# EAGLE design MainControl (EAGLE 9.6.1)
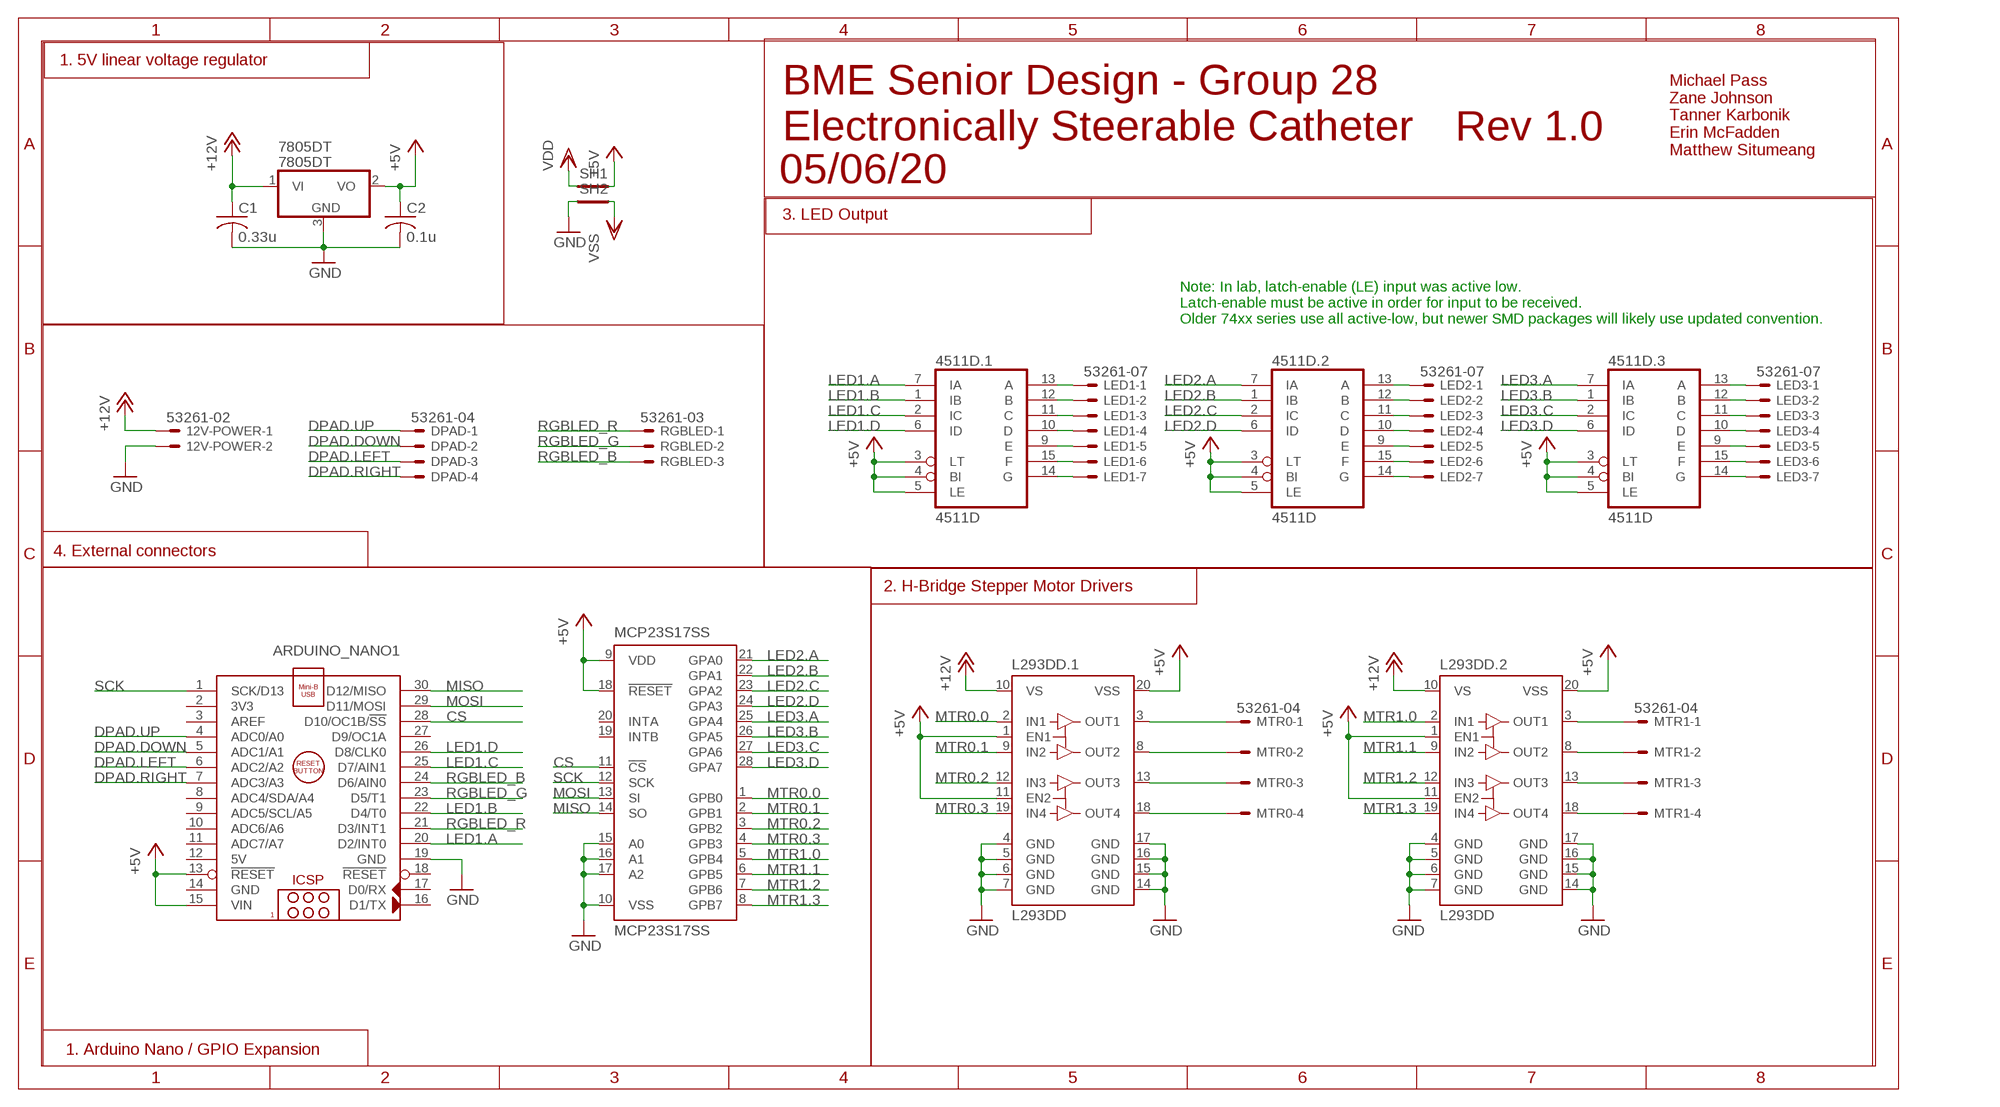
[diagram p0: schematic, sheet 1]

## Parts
12V-POWER  53261-02  [53261-02]
4511D.1  4511D  [SO16]
4511D.2  4511D  [SO16]
4511D.3  4511D  [SO16]
7805DT  7805DT  [TO252]
ARDUINO_NANO1  ARDUINO_NANO  [ARDUINO_NANO]
C1  0.33u  C-USC0805  [C0805]
C2  0.1u  C-USC0805  [C0805]
DPAD  53261-04  [53261-04]
L293DD.1  L293DD  [SO20]
L293DD.2  L293DD  [SO20]
LED1  53261-07  [53261-07]
LED2  53261-07  [53261-07]
LED3  53261-07  [53261-07]
MCP23S17SS  MCP23S17SS  [SSOP28]
MTR0  53261-04  [53261-04]
MTR1  53261-04  [53261-04]
RGBLED  53261-03  [53261-03]
SH1  SHORTT5  [SHORT_TOP-50]
SH2  SHORTT5  [SHORT_TOP-50]

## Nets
+5V: 4511D.1.3(LT) 4511D.1.4(BI) 4511D.1.5(LE) 4511D.2.3(LT) 4511D.2.4(BI) 4511D.2.5(LE) 4511D.3.3(LT) 4511D.3.4(BI) 4511D.3.5(LE) 7805DT.2(VO) ARDUINO_NANO1.13(!RESET) ARDUINO_NANO1.15(VIN) C2.1 L293DD.1.1(EN1) L293DD.1.11(EN2) L293DD.1.20(VSS) L293DD.2.1(EN1) L293DD.2.11(EN2) L293DD.2.20(VSS) MCP23S17SS.9(VDD) MCP23S17SS.18(!RESET) SH1.2
+12V: 12V-POWER.1 7805DT.1(VI) C1.1 L293DD.1.10(VS) L293DD.2.10(VS)
CS: ARDUINO_NANO1.28(D10/OC1B/!SS) MCP23S17SS.11(!CS)
DPAD.DOWN: ARDUINO_NANO1.5(ADC1/A1) DPAD.2
DPAD.LEFT: ARDUINO_NANO1.6(ADC2/A2) DPAD.3
DPAD.RIGHT: ARDUINO_NANO1.7(ADC3/A3) DPAD.4
DPAD.UP: ARDUINO_NANO1.4(ADC0/A0) DPAD.1
GND: 12V-POWER.2 7805DT.3(GND) ARDUINO_NANO1.19(GND) C1.2 C2.2 L293DD.1.4(GND) L293DD.1.5(GND) L293DD.1.6(GND) L293DD.1.7(GND) L293DD.1.14(GND) L293DD.1.15(GND) L293DD.1.16(GND) L293DD.1.17(GND) L293DD.2.4(GND) L293DD.2.5(GND) L293DD.2.6(GND) L293DD.2.7(GND) L293DD.2.14(GND) L293DD.2.15(GND) L293DD.2.16(GND) L293DD.2.17(GND) MCP23S17SS.10(VSS) MCP23S17SS.15(A0) MCP23S17SS.16(A1) MCP23S17SS.17(A2) SH2.1
LED1.A: 4511D.1.7(IA) ARDUINO_NANO1.20(D2/INT0)
LED1.B: 4511D.1.1(IB) ARDUINO_NANO1.22(D4/T0)
LED1.C: 4511D.1.2(IC) ARDUINO_NANO1.25(D7/AIN1)
LED1.D: 4511D.1.6(ID) ARDUINO_NANO1.26(D8/CLK0)
LED2.A: 4511D.2.7(IA) MCP23S17SS.21(GPA0)
LED2.B: 4511D.2.1(IB) MCP23S17SS.22(GPA1)
LED2.C: 4511D.2.2(IC) MCP23S17SS.23(GPA2)
LED2.D: 4511D.2.6(ID) MCP23S17SS.24(GPA3)
LED3.A: 4511D.3.7(IA) MCP23S17SS.25(GPA4)
LED3.B: 4511D.3.1(IB) MCP23S17SS.26(GPA5)
LED3.C: 4511D.3.2(IC) MCP23S17SS.27(GPA6)
LED3.D: 4511D.3.6(ID) MCP23S17SS.28(GPA7)
MISO: ARDUINO_NANO1.30(D12/MISO) MCP23S17SS.14(SO)
MOSI: ARDUINO_NANO1.29(D11/MOSI) MCP23S17SS.13(SI)
MTR0.0: L293DD.1.2(IN1) MCP23S17SS.1(GPB0)
MTR0.1: L293DD.1.9(IN2) MCP23S17SS.2(GPB1)
MTR0.2: L293DD.1.12(IN3) MCP23S17SS.3(GPB2)
MTR0.3: L293DD.1.19(IN4) MCP23S17SS.4(GPB3)
MTR1.0: L293DD.2.2(IN1) MCP23S17SS.5(GPB4)
MTR1.1: L293DD.2.9(IN2) MCP23S17SS.6(GPB5)
MTR1.2: L293DD.2.12(IN3) MCP23S17SS.7(GPB6)
MTR1.3: L293DD.2.19(IN4) MCP23S17SS.8(GPB7)
N$1: 4511D.1.13(A) LED1.1
N$2: 4511D.1.12(B) LED1.2
N$3: 4511D.1.11(C) LED1.3
N$12: 4511D.1.10(D) LED1.4
N$13: 4511D.1.9(E) LED1.5
N$14: 4511D.1.15(F) LED1.6
N$15: 4511D.1.14(G) LED1.7
N$16: 4511D.2.13(A) LED2.1
N$17: 4511D.2.12(B) LED2.2
N$18: 4511D.2.11(C) LED2.3
N$19: 4511D.2.10(D) LED2.4
N$20: 4511D.2.9(E) LED2.5
N$21: 4511D.2.15(F) LED2.6
N$22: 4511D.2.14(G) LED2.7
N$23: 4511D.3.13(A) LED3.1
N$24: 4511D.3.12(B) LED3.2
N$25: 4511D.3.11(C) LED3.3
N$26: 4511D.3.10(D) LED3.4
N$27: 4511D.3.9(E) LED3.5
N$28: 4511D.3.15(F) LED3.6
N$29: 4511D.3.14(G) LED3.7
N$30: L293DD.1.3(OUT1) MTR0.1
N$31: L293DD.1.8(OUT2) MTR0.2
N$32: L293DD.1.13(OUT3) MTR0.3
N$33: L293DD.1.18(OUT4) MTR0.4
N$34: L293DD.2.3(OUT1) MTR1.1
N$35: L293DD.2.8(OUT2) MTR1.2
N$36: L293DD.2.13(OUT3) MTR1.3
N$37: L293DD.2.18(OUT4) MTR1.4
RGBLED_B: ARDUINO_NANO1.24(D6/AIN0) RGBLED.3
RGBLED_G: ARDUINO_NANO1.23(D5/T1) RGBLED.2
RGBLED_R: ARDUINO_NANO1.21(D3/INT1) RGBLED.1
SCK: ARDUINO_NANO1.1(SCK/D13) MCP23S17SS.12(SCK)
VDD: SH1.1
VSS: SH2.2
Unconnected: ARDUINO_NANO1.2(3V3) ARDUINO_NANO1.3(AREF) ARDUINO_NANO1.8(ADC4/SDA/A4) ARDUINO_NANO1.9(ADC5/SCL/A5) ARDUINO_NANO1.10(ADC6/A6) ARDUINO_NANO1.11(ADC7/A7) ARDUINO_NANO1.16(D1/TX) ARDUINO_NANO1.17(D0/RX) ARDUINO_NANO1.18(!RESET) ARDUINO_NANO1.27(D9/OC1A) MCP23S17SS.19(INTB) MCP23S17SS.20(INTA)

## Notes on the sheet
- 1. 5V linear voltage regulator
- BME Senior Design - Group 28
- Electronically Steerable Catheter | Rev 1.0
- Michael Pass
  Zane Johnson
  Tanner Karbonik
  Erin McFadden
  Matthew Situmeang
- 05/06/20
- 3. LED Output
- Note: In lab, latch-enable (LE) input was active low. 
  Latch-enable must be active in order for input to be received. 
  Older 74xx series use all active-low, but newer SMD packages will likely use updated convention.
- 4. External connectors
- 2. H-Bridge Stepper Motor Drivers
- 1. Arduino Nano / GPIO Expansion

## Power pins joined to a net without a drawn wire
5V: ARDUINO_NANO1.12(5V)
GND: ARDUINO_NANO1.14(GND)
VDD: 4511D.1.16(VDD) 4511D.2.16(VDD) 4511D.3.16(VDD)
VSS: 4511D.1.8(VSS) 4511D.2.8(VSS) 4511D.3.8(VSS)

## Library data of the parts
12V-POWER = con-molex:53?-02: CONNECTOR; MF: MOLEX; OC_FARNELL: 1125373; OC_NEWARK: unknown
4511D.1-4511D.3 = 45xx:4511: BCD to 7-segment LATCH/DECODER/DRIVER
7805DT = linear:78*: Positive VOLTAGE REGULATOR Source: http://cache.national.com/ds/LM/LM78L05.pdf http://www.fairchildsemi.com/ds/LM/LM7805.pdf
ARDUINO_NANO1 = ArduinoNanoV30:ARDUINO_NANO: Arduino Nano V3.0 Module Overview: The Arduino Nano is a small, complete, and breadboard-friendly board based on the ATmega328 (Arduino Nano 3.x) or ATmega168 (Arduino Nano 2.x). It has more or less the same functionality of the Arduino Duemilanove, but in a different package. It lacks only a DC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
C1 C2 = rcl:C-US: CAPACITOR, American symbol; SPICEPREFIX: C
DPAD MTR0 MTR1 = con-molex:53?-04: CONNECTOR wire to board 1.25 mm (.049 inch) pitch header; MF: MOLEX; OC_FARNELL: 1125374; OC_NEWARK: unknown
L293DD.1 L293DD.2 = st-microelectronics:L293DD: PUSH-PULL FOUR CHANNEL DRIVER WITH DIODES Source: http://www.st.com/stonline/books/pdf/docs/1330.pdf; OC_FARNELL: unknown
LED1-LED3 = con-molex:53?-07: CONNECTOR wire to board 1.25 mm (.049 inch) pitch header; MF: MOLEX; OC_FARNELL: 1125361; OC_NEWARK: unknown
MCP23S17SS = microchip:MCP23S17: http://ww1.microchip.com/downloads/en/DeviceDoc/21952a.pdf Source: http://ww1.microchip.com/downloads/en/DeviceDoc/21952a.pdf; MF: MICROCHIP; MPN: MCP23S17-E/SS; OC_FARNELL: 1467675; OC_NEWARK: 31K2952
RGBLED = con-molex:53?-03: CONNECTOR wire to board 1.25 mm (.049 inch) pitch header; MF: MOLEX; MPN: 53261-0390; OC_FARNELL: 1125359; OC_NEWARK: 57H5006
SH1 SH2 = shorts:SHORT: Short between two nets; BOM: no

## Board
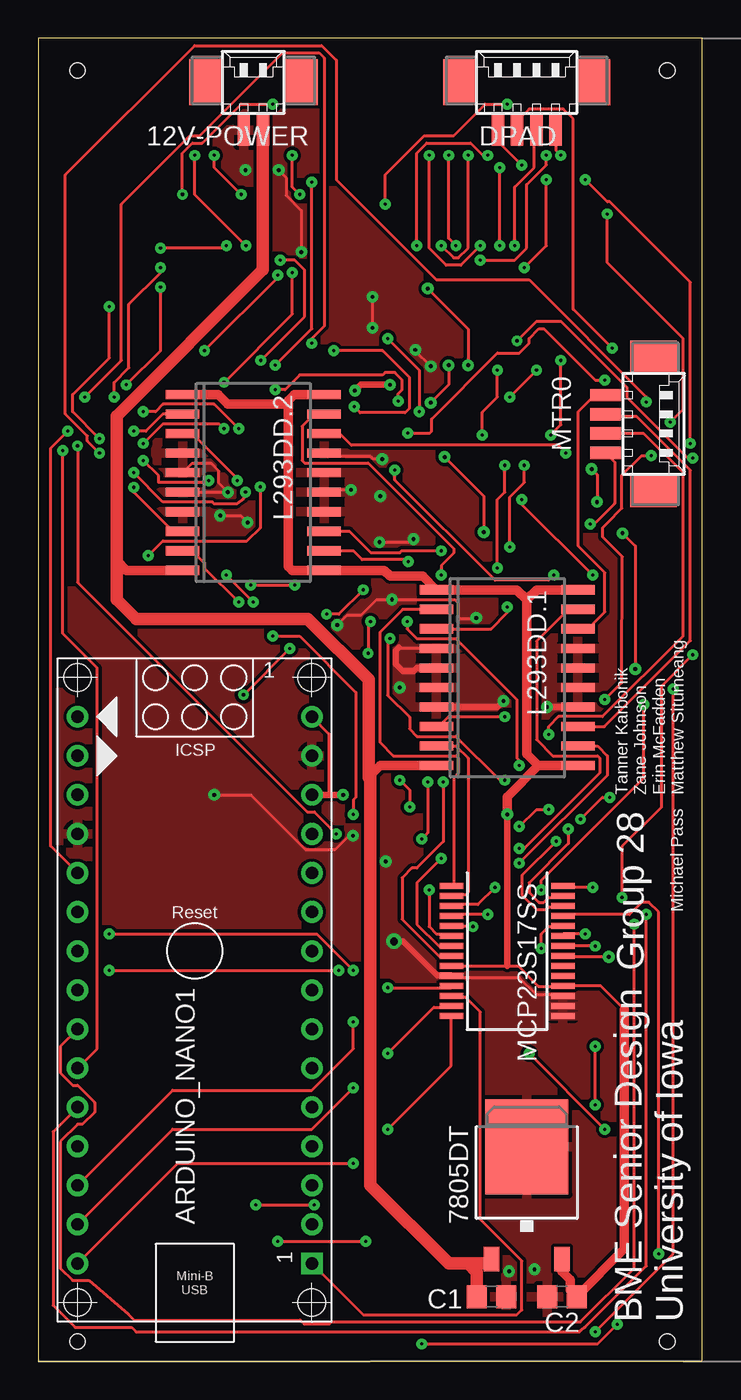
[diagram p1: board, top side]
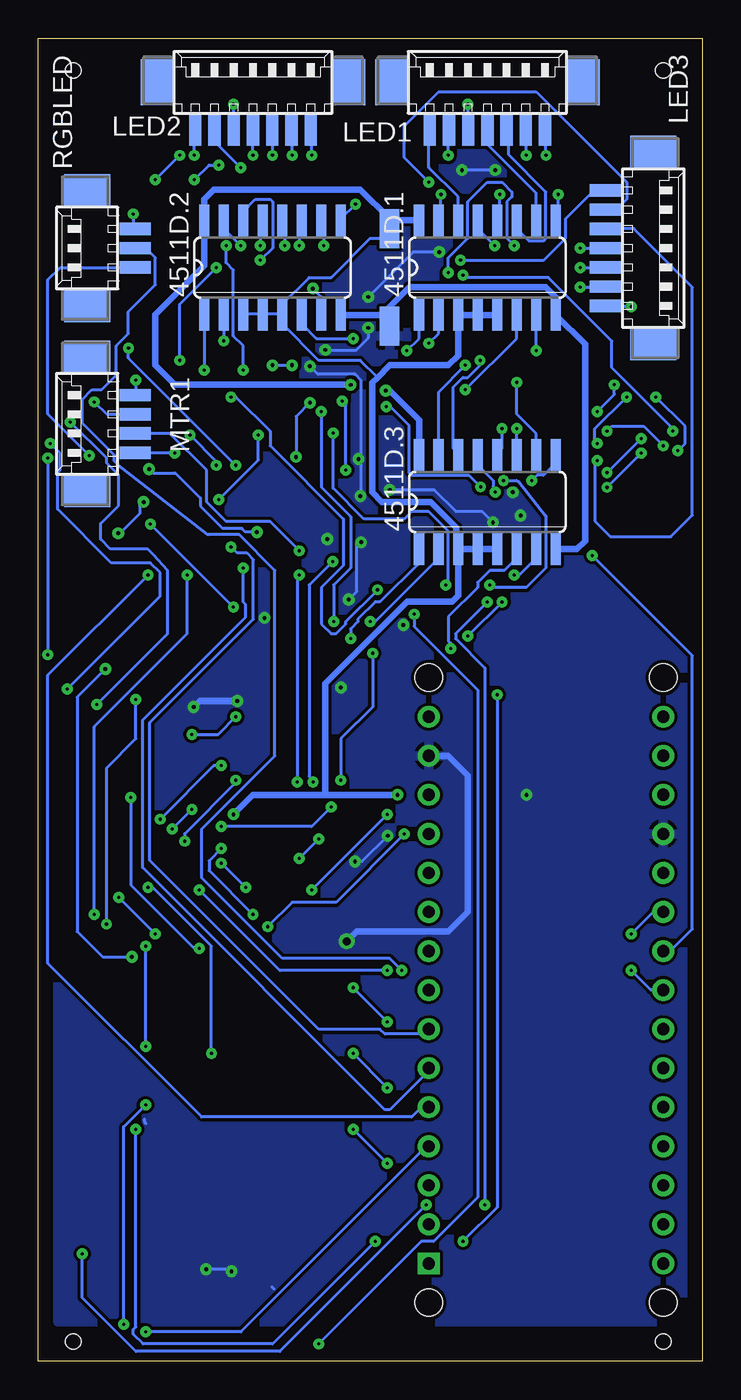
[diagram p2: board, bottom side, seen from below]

Size 43.16 x 86.03 mm. Coordinates in mm from the lower left corner, seen from the top.
Outline: 0,0 43.16,0 43.16,86.03 0,86.03 0,0
Copper layers (1*16): Top 0.035mm / dielectric 1.5mm / Bottom 0.035mm
Design rules "SparkFun *": minimum track width 8mil, minimum drill 0.2mm, track to track 8mil, track to pad 8mil, pad to pad 8mil, via to via 8mil, smd to smd 8mil, copper to edge 10mil, drill to drill 8mil, minimum pad ring 12mil, minimum via ring 10mil, stop-mask expansion 4mil, vias tented up to drill 25mil, thermal gap 10mil
Holes 1 mm at 40.89,83.95 2.54,83.95 2.54,1.27 40.89,1.27

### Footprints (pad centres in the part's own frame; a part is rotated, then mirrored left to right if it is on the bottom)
53261-02 = smd 0.8 x 2: 1 0.625,-2.5; 2 -0.625,-2.5 | smd 2.1 x 3: S1 3.125,0.625; S2 -3.125,0.625
SO16 = smd 0.66 x 2.032: 1 -4.445,-3.073; 2 -3.175,-3.073; 3 -1.905,-3.073; 4 -0.635,-3.073; 5 0.635,-3.073; 6 1.905,-3.073; 7 3.175,-3.073; 8 4.445,-3.073; 9 4.445,3.073; 10 3.175,3.073; 11 1.905,3.073; 12 0.635,3.073; 13 -0.635,3.073; 14 -1.905,3.073; 15 -3.175,3.073; 16 -4.445,3.073
TO252 = smd 1 x 1.6: 1 -2.28,-4.8; 2 2.28,-4.8 | smd 5.4 x 6.2: 3 0,2.5
ARDUINO_NANO = drill 0.8 square: 1 -20.32,-7.62 | drill 0.8: 2 -17.78,-7.62; 3 -15.24,-7.62; 4 -12.7,-7.62; 5 -10.16,-7.62; 6 -7.62,-7.62; 7 -5.08,-7.62; 8 -2.54,-7.62; 9 0,-7.62; 10 2.54,-7.62; 11 5.08,-7.62; 12 7.62,-7.62; 13 10.16,-7.62; 14 12.7,-7.62; 15 15.24,-7.62; 16 15.24,7.62; 17 12.7,7.62; 18 10.16,7.62; 19 7.62,7.62; 20 5.08,7.62; 21 2.54,7.62; 22 0,7.62; 23 -2.54,7.62; 24 -5.08,7.62; 25 -7.62,7.62; 26 -10.16,7.62; 27 -12.7,7.62; 28 -15.24,7.62; 29 -17.78,7.62; 30 -20.32,7.62 | hole 1.778: -22.86,-7.62; -22.86,7.62; 17.78,7.62; 17.78,-7.62
C0805 = smd 1.3 x 1.5: 1 -0.95,0; 2 0.95,0
53261-04 = smd 0.8 x 2: 1 1.875,-2.5; 2 0.625,-2.5; 3 -0.625,-2.5; 4 -1.875,-2.5 | smd 2.1 x 3: S1 4.375,0.625; S2 -4.375,0.625
SO20 = smd 0.6 x 2.2: 1 -5.715,-4.6; 2 -4.445,-4.6; 3 -3.175,-4.6; 4 -1.905,-4.6; 5 -0.635,-4.6; 6 0.635,-4.6; 7 1.905,-4.6; 8 3.175,-4.6; 9 4.445,-4.6; 10 5.715,-4.6; 11 5.715,4.6; 12 4.445,4.6; 13 3.175,4.6; 14 1.905,4.6; 15 0.635,4.6; 16 -0.635,4.6; 17 -1.905,4.6; 18 -3.175,4.6; 19 -4.445,4.6; 20 -5.715,4.6
53261-07 = smd 0.8 x 2: 1 3.75,-2.5; 2 2.5,-2.5; 3 1.25,-2.5; 4 0,-2.5; 5 -1.25,-2.5; 6 -2.5,-2.5; 7 -3.75,-2.5 | smd 2.1 x 3: S1 6.25,0.625; S2 -6.25,0.625
SSOP28 = smd 0.4 x 1.5: 1 -4.225,-3.625; 2 -3.575,-3.625; 3 -2.925,-3.625; 4 -2.275,-3.625; 5 -1.625,-3.625; 6 -0.975,-3.625; 7 -0.325,-3.625; 8 0.325,-3.625; 9 0.975,-3.625; 10 1.625,-3.625; 11 2.275,-3.625; 12 2.925,-3.625; 13 3.575,-3.625; 14 4.225,-3.625; 15 4.225,3.625; 16 3.575,3.625; 17 2.925,3.625; 18 2.275,3.625; 19 1.625,3.625; 20 0.975,3.625; 21 0.325,3.625; 22 -0.325,3.625; 23 -0.975,3.625; 24 -1.625,3.625; 25 -2.275,3.625; 26 -2.925,3.625; 27 -3.575,3.625; 28 -4.225,3.625
53261-03 = smd 0.8 x 2: 1 1.25,-2.5; 2 0,-2.5; 3 -1.25,-2.5 | smd 2.1 x 3: S1 3.75,0.625; S2 -3.75,0.625
SHORT_TOP-50 = smd 1.27 x 1.27: 1 0.635,0; 2 -0.635,0

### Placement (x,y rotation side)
12V-POWER  13.97,82.55 0 top
4511D.1  13.97,71.12 0 bottom
4511D.2  27.94,71.12 0 bottom
4511D.3  13.97,55.88 0 bottom
7805DT  31.75,11.43 0 top
ARDUINO_NANO1  10.16,26.67 90 top
C1  29.46,4.19 0 top
C2  34.04,4.19 180 top
DPAD  31.75,82.55 0 top
L293DD.1  30.48,44.45 270 top
L293DD.2  13.97,57.15 270 top
LED1  13.97,82.55 0 bottom
LED2  29.21,82.55 0 bottom
LED3  3.81,72.39 270 bottom
MCP23S17SS  30.48,26.67 270 top
MTR0  39.37,60.96 270 top
MTR1  39.37,60.96 90 bottom
RGBLED  39.37,72.39 90 bottom
SH1  20.32,73.66 90 bottom
SH2  20.32,67.31 270 bottom

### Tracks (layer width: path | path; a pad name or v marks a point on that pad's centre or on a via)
+5V  (via drill 0.25)
  Top 0.203: 38.1,22.86 36.56,24.39 MCP23S17SS.18 34.09,24.38 32.51,24.38 31.2,25.7 30.48,25.7 MCP23S17SS.9 | L293DD.2.20 18.03,62.87 | 18.89,36.83 18.89,40.8 ARDUINO_NANO1.15
  Top 0.406: ARDUINO_NANO1.13 18.89,36.83 v19.81,36.83 | v30.48,35.56 30.48,25.7
  Top 0.61: 7805DT.2 34.03,5.84 34.58,5.29 34.58,4.6 C2.1 38.1,7.3 38.1,22.86 | v30.48,35.56 30.48,36.7 32.51,38.73 | 32.51,38.73 L293DD.1.11 | 32.51,38.73 31.75,39.5 31.75,49.53 | 31.75,49.53 32.38,50.16 L293DD.1.20 | 31.75,49.53 31.11,50.16 L293DD.1.1 24.99,51.05 22.86,51.05 22.48,51.44 L293DD.2.11 16.51,51.44 16.26,51.69 16.26,62.23 | 16.26,62.23 16.26,62.48 16.64,62.87 18.03,62.87 | 16.26,62.23 12.32,62.23 11.68,62.87 L293DD.2.1
  Bottom 0.203: SH1.2 21.59,73.03 24.13,70.48 25.56,70.48 27.3,68.74 27.3,68.1 | 27.3,68.1 28.57,68.1 | 27.3,68.1 4511D.2.5 27.3,67.47 24.92,65.09 22.23,65.09 21.11,63.98 | 28.57,68.1 29.84,68.1 4511D.2.3 | 28.57,68.1 4511D.2.4
  Bottom 0.406: v19.81,36.83 24.51,36.83 | 24.51,36.83 29.21,36.83 v30.48,35.56 | 24.51,36.83 24.51,44.07 19.18,49.4 16.26,49.4 15.88,49.78 4511D.3.3 | 4511D.3.3 4511D.3.4 4511D.3.5 | 4511D.3.3 16,52.93 16,54.23 17.65,55.88 20.83,55.88 21.46,56.52 21.46,63.63 21.11,63.98 20.32,64.77 16.51,64.77 15.88,65.41 4511D.1.3 4511D.1.4 4511D.1.5
+12V
  Top 0.61: L293DD.2.10 5.71,51.44 5.08,52.07 | 21.46,37.97 21.59,38.1 22.23,38.73 L293DD.1.10
  Top 0.813: 12V-POWER.1 14.6,70.98 5.08,61.47 5.08,52.07 5.08,49.53 6.35,48.26 17.53,48.26 21.46,44.32 21.46,37.97 | 27.94,6.35 26.67,6.35 21.59,11.43 21.59,38.1 | 27.94,6.35 29.19,6.35 7805DT.1 | 27.94,6.35 28.51,5.78 C1.1
CS  (via drill 0.2)
  Top 0.203: v22.7,24.29 26.83,24.29 MCP23S17SS.11 | v20.48,22.07 20.48,20.32 17.78,17.62 8.73,17.62 ARDUINO_NANO1.28
  Bottom 0.203: v20.48,22.07 v22.7,24.29
DPAD.DOWN  (via drill 0.2)
  Top 0.203: v30.96,72.55 30.96,76.36 32.23,77.63 32.23,80.01 DPAD.2 | v29.84,64.45 29.84,62.71 28.86,61.72 v28.86,60.23 | v31.43,56.04 31.43,55.72 v36.04,51.12
  Bottom 0.203: v30.96,72.55 30.96,71.44 30.48,70.96 30.48,66.67 29.84,66.04 v29.84,64.45 | v28.86,60.23 28.86,58.61 v31.43,56.04 | v36.04,51.12 42.55,44.61 42.55,25.88 32.54,15.88 18.89,15.88 18.26,16.51 ARDUINO_NANO1.5
DPAD.LEFT  (via drill 0.2)
  Top 0.203: v37.31,65.88 34.77,68.42 34.77,80.8 34.13,81.44 31.91,81.44 31.27,80.8 31.27,80.17 DPAD.3 | v30.32,58.26 30.32,56.52 29.84,56.04 v29.84,51.59
  Bottom 0.203: v37.31,65.88 37.31,65.25 v30.32,58.26 | v29.84,51.59 29.84,49.37 29.69,49.21 29.69,48.39 36.39,41.69 36.39,32.1 20.64,16.35 20.32,16.35 17.78,18.89 ARDUINO_NANO1.6
DPAD.RIGHT  (via drill 0.2)
  Top 0.203: v31.43,77.79 30,79.22 30,80.01 DPAD.4 | v33.02,76.83 33.02,72.55 v31.59,71.12 | v33.97,65.09 33.97,60.9 v33.31,60.23 | v31.59,58.26 31.59,57.15 30.64,56.2 v30.64,52.96
  Bottom 0.203: v31.43,77.79 32.07,77.79 v33.02,76.83 | v31.59,71.12 33.97,68.74 v33.97,65.09 | v31.59,58.26 31.59,58.52 v33.31,60.23 | v30.64,52.96 30.26,52.58 29.62,52.58 29.18,52.13 29.18,48.26 35.91,41.53 35.91,32.58 24.92,21.59 20.95,21.59 20.64,21.27 18.1,21.27 ARDUINO_NANO1.7
DPAD.UP  (via drill 0.2)
  Top 0.203: v33.97,78.42 33.66,78.74 33.66,80.01 DPAD.1 | v35.56,76.83 36.99,75.41 37.15,75.41 42.39,70.17 v42.39,59.69 | v41.27,43.72 41.27,6.99 v36.2,1.91
  Bottom 0.203: v35.56,76.83 v33.97,78.42 | v42.39,59.69 41.75,59.05 41.75,57.94 41.91,57.78 41.91,55.4 38.42,51.91 35.88,51.91 35.24,51.28 35.24,49.75 v41.27,43.72 | v36.2,1.91 30,1.91 17.94,13.97 ARDUINO_NANO1.4
GND  (via drill 0.25, 0.51)
  Top 0.203: MCP23S17SS.10 26.99,24.92 31.27,24.92 32.38,23.81 33.97,23.81 MCP23S17SS.17 | v25.51,64.71 24.51,65.71 v24.51,65.77 | v22.35,58.67 21.75,58.67 21.6,58.83 18.8,58.83 L293DD.2.17 | L293DD.1.4 23.49,46.35 23.43,46.42 | v19.43,47.88 20.07,48.52 20.97,48.52 21.98,49.53 v22.99,49.53 27.08,49.53 27.29,49.32 27.29,48.38 27.38,48.28 28.41,48.28 v28.46,48.34 | v15.62,77.47 16.1,76.99 16.1,75.83 17.1,74.84 v17.1,72.14 | v21.72,69.22 v21.72,67.2 | v11.81,54.99 13.16,54.99 v13.6,54.55 | v20.32,56.66 18.72,56.66 L293DD.2.15 | L293DD.2.6 v12.32,56.52 11.74,57.09 11.74,57.88 11.25,58.37 9.96,58.37 L293DD.2.5 | v11.43,36.83 13.81,36.83 17.36,33.28 19.29,33.28 20.18,34.17 v20.45,34.17 | v22.18,53.26 24.18,53.26 v24.38,53.47
  Top 0.406: MCP23S17SS.10 26.81,25.09 25.94,25.09 23.72,27.3 v23.11,27.3 | 23.43,46.42 23.24,46.23 23.24,45.34 23.68,44.9 24.41,44.9 24.6,45.09 L293DD.1.5 | L293DD.1.7 29.84,42.55 v30.23,42.94 | v33.07,42.55 L293DD.1.14
  Bottom 0.203: v25.51,64.71 24.99,64.18 22.58,64.18 22.18,63.78 22.18,56.31 v22.23,56.26 | v24.51,65.77 22.49,65.77 21.72,66.55 v21.72,67.2 | v30.61,5.84 30.73,5.97 v32.26,5.97 | v13.46,77.47 v15.62,77.47 | v17.1,72.14 18.8,72.14 v21.72,69.22 | v13.6,54.55 14.3,55.24 16,55.24 17.42,56.66 v20.32,56.66 | 36.17,15.44 36.27,15.74 | 27.84,4.67 27.97,4.8 | v20.45,34.17 22.13,32.49 v22.58,32.49 | v22.99,49.53 22.45,50.06 22.45,53.34 22.25,53.34 v22.18,53.26
  Bottom 0.406: v23.11,27.3 22.48,27.94 16.51,27.94 15.24,29.21 15.24,38.1 16.51,39.37 ARDUINO_NANO1.14 | v30.23,42.94 32.68,42.94 v33.07,42.55
  other vias: 23.5,43.81
  pour Top: 1.27,85.09 41.91,85.09 41.91,2.54 1.27,2.54
  pour Bottom: 1.27,85.09 41.91,85.09 41.91,2.54 1.27,2.54
LED1.A  (via drill 0.2)
  Top 0.203: v10.79,65.72 15.56,70.48 v15.56,70.64 | v1.91,60.48 0.79,59.37 0.79,33.5 ARDUINO_NANO1.20
  Bottom 0.203: v10.79,65.72 4511D.1.7 | v15.56,70.64 15.4,70.48 10,70.48 5.87,66.36 5.87,64.61 1.91,60.64 v1.91,60.48
LED1.B  (via drill 0.2)
  Top 0.203: v19.21,65.72 22.38,65.72 24.13,63.98 24.13,61.98 23.84,61.69 20.92,61.69 v20.54,62.07 | v14.41,56.86 14.41,54.2 13.56,53.34 8.1,53.34 v7.14,52.39
  Bottom 0.203: 4511D.1.1 18.41,66.52 v19.21,65.72 | v20.54,62.07 20.29,62.07 19.05,60.83 19.05,57.78 18.89,57.63 15.18,57.63 v14.41,56.86 | v7.14,52.39 0.64,45.88 0.64,28.1 2.06,26.67 ARDUINO_NANO1.22
LED1.C  (via drill 0.2)
  Top 0.203: v17.78,66.2 17.78,66.52 18.57,67.31 18.57,84.77 18.26,85.09 15.88,85.09 10.48,79.69 9.84,79.69 5.4,75.25 5.4,65.09 v3.02,62.71 | v1.59,59.21 1.59,47.31 3.81,45.09 3.81,20.32 ARDUINO_NANO1.25
  Bottom 0.203: 4511D.1.2 17.14,66.83 v17.78,66.2 | v3.02,62.71 1.11,60.8 1.11,59.69 v1.59,59.21
LED1.D  (via drill 0.2)
  Top 0.203: v15.4,63.18 16.03,63.18 16.99,64.14 22.38,64.14 22.54,64.29 23.18,64.29 23.65,63.82 23.65,63.18 23.4,62.93 v23.4,62.45 | v23.18,57.94 23.18,57.31 29.69,50.8 33.18,50.8 v33.5,51.12 | v39.53,29.05 39.53,6.19 35.53,2.19 35.18,1.91 6.35,1.91 6.06,2.19 2.38,2.19 0.95,3.62 0.95,14.92 ARDUINO_NANO1.26
  Bottom 0.203: 4511D.1.6 12.06,66.52 v15.4,63.18 | v23.4,62.45 23.18,62.23 v23.18,57.94 | v33.5,51.12 33.5,47.31 39.53,41.27 v39.53,29.05
LED2.A  (via drill 0.25)
  Top 0.203: v25.31,69.76 27.94,67.14 v27.94,64.77 | v26.67,64.77 26.67,63.5 v25.51,62.34 | v26.41,58.81 28.96,56.26 v28.96,53.93 | v35.97,58.02 36.32,57.66 v36.32,55.88 | v37.97,53.85 38.81,53.01 v38.81,45.01 | v37.08,26.29 34.16,26.29 MCP23S17SS.21
  Bottom 0.203: 4511D.2.7 24.77,69.22 v25.31,69.76 | v27.94,64.77 v26.67,64.77 | v25.51,62.34 26.41,61.43 v26.41,58.81 | v28.96,53.93 29.7,53.93 29.93,54.16 31.17,54.16 32.64,55.63 32.64,56.13 34.27,57.76 35.71,57.76 v35.97,58.02 | v36.32,55.88 36.58,55.63 36.58,55.12 36.96,54.74 37.08,54.61 37.85,53.85 v37.97,53.85 | v38.81,45.01 40.64,43.18 40.64,27.94 38.99,26.29 v37.08,26.29
LED2.B  (via drill 0.2)
  Top 0.203: v36.2,26.99 34.13,26.99 MCP23S17SS.22 | v36.2,16.67 v36.2,20.48 | v37.62,2.38 36.35,1.11 v24.92,1.11 | v18.73,48.58 19.53,48.58 v21.11,50.16 | v32.38,64.45 v30.64,62.71
  Bottom 0.203: v36.2,20.48 v36.2,26.99 | v36.2,16.67 37.62,15.24 v37.62,2.38 | v24.92,1.11 18.26,7.78 17.46,7.78 14.61,10.64 14.61,43.66 18.73,47.78 v18.73,48.58 | v21.11,50.16 23.18,48.1 23.18,47.94 23.81,47.31 24.13,47.31 24.77,47.94 24.77,50.32 23.34,51.75 23.34,54.77 28.1,59.53 28.1,60.48 30.32,62.71 v30.64,62.71 | 4511D.2.1 v32.38,64.45
LED2.C  (via drill 0.2)
  Top 0.203: v35.56,27.78 34.13,27.78 MCP23S17SS.23 | v37.94,30.16 37.94,33.47 40.48,36.01 40.48,43.88 v42.55,45.94 | v42.55,58.74 42.23,58.74 38.26,62.71 38.26,63.34 33.97,67.63 32.38,67.63 v31.11,66.36
  Bottom 0.203: v37.94,30.16 v35.56,27.78 | v42.55,58.74 v42.55,45.94 | 4511D.2.2 v31.11,66.36
LED2.D  (via drill 0.2)
  Top 0.203: v32.7,26.83 32.7,27.78 33.18,28.26 33.97,28.26 MCP23S17SS.24 | v37.15,36.67 36.67,36.67 v35.24,35.24 | v31.27,38.73 31.27,39.05 31.11,39.21 31.11,43.02 27.15,46.99 24.61,46.99 23.97,47.62 v23.97,48.1 | v24.77,61.75 24.77,64.45 v22.7,66.52
  Bottom 0.203: v32.7,26.83 33.02,26.83 37.15,30.96 v37.15,36.67 | v35.24,35.24 31.75,38.73 v31.27,38.73 | v23.97,48.1 23.97,50.48 22.86,51.59 22.86,54.93 24.77,56.83 v24.77,61.75 | v22.7,66.52 25.08,66.52 26.04,67.47 4511D.2.6
LED3.A  (via drill 0.2)
  Top 0.203: v40.32,6.99 40.32,29.21 39.69,29.84 39.21,29.84 38.42,29.05 34.13,29.05 MCP23S17SS.25 | v14.13,10.16 v17.94,10.16 | v12.22,51.12 v13.97,49.37
  Bottom 0.203: v40.32,6.99 40.32,4.13 36.83,0.64 27.46,0.64 v17.94,10.16 | v14.13,10.16 14.13,45.09 16.03,46.99 16.03,47.31 v13.97,49.37 | v12.22,51.12 11.91,51.12 10.79,52.23 4511D.3.7
LED3.B  (via drill 0.2)
  Top 0.203: v33.66,33.81 31.43,31.59 31.43,30.32 32.38,29.37 33.02,29.37 33.18,29.53 33.97,29.53 MCP23S17SS.26 | v30.32,37.78 30,37.78 27.15,40.64 24.61,40.64 24.13,41.12 24.13,41.88 22.7,43.31 22.7,46.83 v22.86,46.99
  Bottom 0.203: v33.66,33.81 33.66,34.29 30.32,37.62 v30.32,37.78 | v22.86,46.99 22.86,47.62 22.38,48.1 22.38,48.26 21.27,49.37 20.95,49.37 18.41,51.91 4511D.3.1
LED3.C  (via drill 0.2)
  Top 0.203: v34.45,34.61 34.45,33.66 31.91,31.11 31.91,30.48 32.54,29.84 32.86,29.84 33.18,30.16 33.97,30.16 MCP23S17SS.27 | v33.18,35.88 32.38,35.88 v31.27,34.77 | v24.13,36.04 24.13,37.15 v23.5,37.78 | v21.43,46.04 21.43,47.94 v21.59,48.1
  Bottom 0.203: v33.18,35.88 v34.45,34.61 | v31.27,34.77 25.4,34.77 v24.13,36.04 | v23.5,37.78 23.5,40.48 21.43,42.55 v21.43,46.04 | v21.59,48.1 21.27,48.1 17.14,52.23 4511D.3.2
LED3.D  (via drill 0.2)
  Top 0.203: v36.04,30.8 34.13,30.8 MCP23S17SS.28 | v36.83,15.08 v31.91,20 | v15.56,7.78 v21.27,7.78 | v16.35,46.35 v13.34,43.34
  Bottom 0.203: v36.04,30.8 35.72,30.8 31.91,26.99 v31.91,20 | v36.83,15.08 36.83,2.22 36.99,2.06 36.99,1.75 36.35,1.11 27.94,1.11 v21.27,7.78 | v15.56,7.78 13.34,10 v13.34,43.34 | v16.35,46.35 16.35,46.67 16.51,46.83 16.51,48.42 14.61,50.32 14.61,50.64 13.81,51.44 12.86,51.44 12.06,52.23 4511D.3.6
MISO  (via drill 0.2)
  Top 0.203: v22.7,15.08 26.83,19.21 26.83,22.38 MCP23S17SS.14 | v20.48,12.86 9.05,12.86 ARDUINO_NANO1.30
  Bottom 0.203: v20.48,12.86 v22.7,15.08
MOSI  (via drill 0.2)
  Top 0.203: v22.7,20 25.72,23.02 26.83,23.02 MCP23S17SS.13 | v20.48,17.78 17.78,15.08 8.73,15.08 ARDUINO_NANO1.29
  Bottom 0.203: v20.48,17.78 v22.7,20
MTR0.0
  Top 0.203: L293DD.1.2 23.69,48.9 22.19,47.4 22.19,40.26 23.08,39.37 27.15,39.37 27.3,39.21 27.3,38.26 26.99,37.94 26.99,30.96 MCP23S17SS.1
MTR0.1
  Top 0.203: L293DD.1.9 27.15,40.01 27.94,39.21 27.94,30.48 27.78,30.32 26.99,30.32 MCP23S17SS.2
MTR0.2  (via drill 0.2)
  Top 0.203: v29.69,30.8 28.57,29.69 26.99,29.69 MCP23S17SS.3 | v31.27,32.38 36.99,38.1 36.99,39.37 36.35,40.01 L293DD.1.12
  Bottom 0.203: v31.27,32.38 v29.69,30.8
MTR0.3  (via drill 0.2)
  Top 0.203: v29.21,29.05 26.99,29.05 MCP23S17SS.4 | v31.27,33.34 31.59,33.34 36.51,38.26 36.51,39.21 36.35,39.37 33.43,39.37 32.38,40.42 32.38,46.83 34.45,48.9 L293DD.1.19
  Bottom 0.203: v29.21,29.05 32.07,31.91 32.07,32.54 v31.27,33.34
MTR1.0  (via drill 0.2)
  Top 0.203: v28.26,28.26 26.99,28.26 MCP23S17SS.5 | v19.37,34.29 17.94,35.72 17.46,35.72 2.54,50.64 v2.54,59.53 | v6.19,60.48 6.99,60.48 8.1,61.59 L293DD.2.2
  Bottom 0.203: v28.26,28.26 26.67,29.84 23.81,29.84 v19.37,34.29 | v2.54,59.53 3.81,60.8 5.87,60.8 v6.19,60.48
MTR1.1  (via drill 0.2)
  Top 0.203: v25.4,30.64 25.4,28.26 25.88,27.78 26.83,27.78 MCP23S17SS.6 | v20.48,35.56 20.48,36.51 20.64,36.67 20.64,43.5 16.99,47.15 v15.24,47.15 | v13.02,49.37 10.79,51.59 10.79,51.91 10,52.7 L293DD.2.9
  Bottom 0.203: v20.48,35.56 v25.4,30.64 | v13.02,49.37 v15.24,47.15
MTR1.2  (via drill 0.2)
  Top 0.203: v26.19,32.7 24.61,31.11 24.61,28.42 26.04,26.99 26.83,26.99 MCP23S17SS.7 | v25.3,37.66 25.3,34.35 v24.92,33.97 | v24.04,52.01 23.91,52.13 21.05,52.13 20.48,52.7 L293DD.2.12
  Bottom 0.203: v24.92,33.97 v26.19,32.7 | v25.3,37.66 25.3,37.78 25.56,38.04 25.56,50.48 v24.04,52.01
MTR1.3  (via drill 0.2)
  Top 0.203: v26.32,37.66 26.32,33.78 24.61,32.07 24.29,32.07 23.65,31.43 23.65,28.73 26.04,26.35 26.83,26.35 MCP23S17SS.8 | v26.19,51.12 26.19,51.75 26.99,52.55 26.99,52.86 21.43,58.42 17.3,58.42 17.14,58.58 17.14,60.8 17.94,61.59 L293DD.2.19
  Bottom 0.203: v26.19,51.12 26.32,50.99 v26.32,37.66
N$1  (via drill 0.2)
  Top 0.203: v10.16,78.42 10.16,75.88 v13.49,72.55
  Bottom 0.203: v10.16,78.42 10.16,80.01 LED1.1 | v13.49,72.55 14.61,73.66 4511D.1.13
N$2  (via drill 0.2)
  Top 0.203: v11.43,78.42 11.43,77.63 v13.18,75.88
  Bottom 0.203: v11.43,78.42 11.43,80.01 LED1.2 | v13.18,75.88 13.18,74.45 13.34,74.3 4511D.1.12
N$3
  Bottom 0.203: 4511D.1.11 12.06,73.66 11.27,72.87 10.32,72.87 10.16,73.03 10.16,76.04 12.57,78.45 12.57,79.76 LED1.3
N$12
  Bottom 0.203: LED1.4 13.97,79.15 10.79,75.98 4511D.1.10
N$13  (via drill 0.2)
  Top 0.203: v15.24,81.76 13.18,81.76 10.64,79.22 10,79.22 9.37,78.58 v9.37,75.88
  Bottom 0.203: v15.24,81.76 15.24,80.17 LED1.5 | v9.37,75.88 9.37,74.45 9.53,74.3 4511D.1.9
N$14  (via drill 0.2)
  Top 0.203: v16.51,78.42 16.51,76.36 v16.99,75.88
  Bottom 0.203: v16.51,78.42 16.51,80.01 LED1.6 | v16.99,75.88 16.99,74.45 17.14,74.3 4511D.1.15
N$15
  Bottom 0.203: 4511D.1.14 15.88,75.72 17.78,77.63 17.78,80.01 LED1.7
N$16  (via drill 0.2)
  Top 0.203: v25.4,78.42 25.4,72.39 26.51,71.28 27.46,71.28 v28.73,72.55
  Bottom 0.203: v25.4,78.42 25.4,80.01 LED2.1 | v28.73,72.55 28.73,73.98 28.57,74.14 4511D.2.13
N$17  (via drill 0.2)
  Top 0.203: v26.67,78.42 26.67,73.03 v27.15,72.55
  Bottom 0.203: v26.67,78.42 26.67,80.01 LED2.2 | v27.15,72.55 27.15,73.98 27.3,74.14 4511D.2.12
N$18  (via drill 0.2)
  Top 0.203: v27.94,78.42 27.94,72.39 27.3,71.75 26.99,71.75 v26.19,72.55
  Bottom 0.203: v27.94,78.42 27.94,80.01 LED2.3 | v26.19,72.55 26.19,73.98 26.04,74.14 4511D.2.11
N$19  (via drill 0.2)
  Top 0.203: v29.21,78.42 28.89,78.42 28.1,79.22 25.24,79.22 24.61,78.58 v24.61,72.55
  Bottom 0.203: v29.21,78.42 LED2.4 | v24.61,72.55 24.61,73.98 24.77,74.14 4511D.2.10
N$20  (via drill 0.2)
  Top 0.203: v30.48,81.76 29.05,81.76 26.99,79.69 25.08,79.69 22.54,77.15 v22.54,75.25
  Bottom 0.203: v30.48,81.76 30.48,80.17 LED2.5 | v22.54,75.25 23.5,74.3 4511D.2.9
N$21  (via drill 0.2)
  Top 0.203: v30,72.55 v30,77.63
  Bottom 0.203: v30,77.63 31.59,79.22 31.59,80.01 LED2.6 | v30,72.55 31.11,73.66 4511D.2.15
N$22  (via drill 0.2)
  Top 0.203: v33.02,78.42 33.02,77.79 31.75,76.52 31.75,72.39 30.96,71.6 v28.73,71.6
  Bottom 0.203: v33.02,78.42 33.02,80.01 LED2.7 | v28.73,71.6 27.94,72.39 27.94,75.41 28.1,75.56 29.05,75.56 29.84,74.77 4511D.2.14
N$23  (via drill 0.2)
  Top 0.203: v4.6,68.58 4.6,65.25 2.22,62.87 2.22,61.75 v3.97,60.01 | v6.19,57.78 8.1,55.88 11.3,55.88 11.43,55.75 12.87,55.75 13.34,56.11 v13.46,56.52
  Bottom 0.203: v4.6,68.58 6.19,68.58 LED3.1 | v6.19,57.78 v3.97,60.01 | v13.46,56.52 13.46,56.77 13.59,56.9 13.59,57.28 14.61,58.29 4511D.3.13
N$24  (via drill 0.2)
  Top 0.203: v7.94,69.85 7.94,65.72 v5.71,63.5 | v6.83,61.75 7.62,61.75 8.1,62.23 11.43,62.23 v13.02,60.64
  Bottom 0.203: v7.94,69.85 6.35,69.85 LED3.2 | v5.71,63.5 5.71,62.87 v6.83,61.75 | v13.02,60.64 13.02,59.37 13.34,59.05 4511D.3.12
N$25  (via drill 0.2)
  Top 0.203: v7.94,71.12 7.94,70.8 5.87,68.74 5.87,64.61 4.92,63.66 v4.92,62.71 | v6.83,59.69 8.1,60.96 11.75,60.96 v12.06,60.64
  Bottom 0.203: v7.94,71.12 6.35,71.12 LED3.3 | v4.92,62.71 6.99,60.64 6.99,59.85 v6.83,59.69 | 4511D.3.11 v12.06,60.64
N$26  (via drill 0.2)
  Top 0.203: v7.94,72.39 12.06,72.39 v12.22,72.55 | v16.51,70.8 16.51,68.1 v12.06,63.66
  Bottom 0.203: v7.94,72.39 LED3.4 | v12.22,72.55 12.7,73.03 12.7,75.41 12.38,75.72 12.38,76.04 13.02,76.68 13.97,76.68 15.24,75.41 15.24,73.03 16.51,71.75 v16.51,70.8 | v12.06,63.66 12.06,61.59 10.79,60.33 4511D.3.10
N$27  (via drill 0.2)
  Top 0.203: v6.83,58.58 7.81,57.59 7.81,57.15 10.95,57.15 v11.08,57.28
  Bottom 0.203: v6.83,58.58 6.99,58.42 6.99,54.64 5.97,53.63 2.03,53.63 0.64,55.02 0.64,69.85 4.45,73.66 6.19,73.66 LED3.5 | v11.08,57.28 10.73,57.63 10.32,57.63 9.53,58.42 4511D.3.9
N$28  (via drill 0.2)
  Top 0.203: v17.78,76.68 17.78,67.15 v15.4,64.77
  Bottom 0.203: v17.78,76.68 19.37,78.26 19.37,80.33 17.14,82.55 10.79,82.55 4.92,76.68 4.92,75.56 5.56,74.93 6.19,74.93 LED3.6 | v15.4,64.77 17.14,63.02 4511D.3.15
N$29  (via drill 0.2)
  Top 0.203: v15.72,71.6 16.67,71.6 17.3,70.96 17.3,67.94 v14.45,65.09
  Bottom 0.203: v15.72,71.6 10.32,71.6 8.89,73.03 8.89,74.3 7.14,76.04 6.35,76.04 LED3.7 | v14.45,65.09 14.45,64.77 15.24,63.98 15.56,63.98 16.19,63.34 16.19,59.37 15.88,59.05 4511D.3.14
N$30  (via drill 0.2)
  Top 0.203: MTR0.1 37.47,58.49 37.47,55.78 36.13,54.45 v35.88,54.45 | v30.48,49.05 30.48,48.67 29.43,47.62 L293DD.1.3
  Bottom 0.203: v30.48,49.05 v35.88,54.45
N$31  (via drill 0.2)
  Top 0.203: v33.18,40.77 33.18,41.27 33.81,41.91 36.67,41.91 41.91,47.15 41.91,57.78 39.37,60.33 36.99,60.33 MTR0.2 | v30.32,41.91 26.67,41.91 26.04,41.27 L293DD.1.8
  Bottom 0.203: v33.18,40.77 31.46,40.77 v30.32,41.91
N$32
  Top 0.203: L293DD.1.13 36.8,41.27 42.39,46.86 42.39,57.94 38.89,61.44 36.99,61.44 MTR0.3
N$33
  Top 0.203: L293DD.1.18 35.72,47.62 36.83,48.74 36.83,51.28 35.08,53.02 35.08,61.75 36.04,62.71 36.83,62.71 MTR0.4
N$34  (via drill 0.2)
  Top 0.203: v36.83,63.82 36.2,63.82 32.86,67.15 32.54,67.15 31.91,66.52 31.91,66.2 31.27,65.56 29.84,65.56 25.56,61.28 25.56,60.48 25.43,60.36 v24,60.36 | v13.81,50.48 v16.67,50.48 | v12.92,57.28 12.92,57.4 10,60.33 L293DD.2.3
  Bottom 0.203: v36.83,63.82 36.83,62.87 MTR1.1 | v24,60.36 24,56.77 22,54.77 19.37,54.77 18.89,55.24 17.78,55.24 16.51,53.98 16.51,50.64 v16.67,50.48 | v13.81,50.48 13.65,50.32 11.43,50.32 10.16,51.59 10.16,54.97 11.93,57.21 12,57.21 12.06,57.28 v12.92,57.28
N$35  (via drill 0.2)
  Top 0.203: v39.53,62.39 39.53,62.71 31.91,70.33 25.88,70.33 19.37,76.83 19.37,84.61 18.41,85.57 10.16,85.57 1.75,77.15 1.75,61.59 3.17,60.17 3.17,59.85 v3.97,59.05 | v6.19,56.83 6.19,56.52 8.73,53.98 L293DD.2.8
  Bottom 0.203: v39.53,62.39 38.73,61.59 36.99,61.59 MTR1.2 | v6.19,56.83 v3.97,59.05
N$36  (via drill 0.2)
  Top 0.203: v26.19,52.7 23.62,52.7 23.5,52.58 21.62,52.58 20.23,53.98 L293DD.2.13
  Bottom 0.203: v26.19,52.7 28.1,54.61 30.96,54.61 32.23,55.88 32.23,57.94 34.61,60.33 36.83,60.33 MTR1.3
N$37  (via drill 0.2)
  Top 0.203: v34.29,59.05 33.78,59.56 20.35,59.56 19.59,60.33 L293DD.2.18
  Bottom 0.203: v34.29,59.05 36.83,59.05 MTR1.4
RGBLED_B  (via drill 0.2)
  Top 0.203: v39.85,58.9 39.21,58.9 37.94,57.63 37.94,55.47 36.96,54.48 36.7,54.23 36.7,53.59 37.97,52.32 37.94,44.13 v36.83,43.02 | v38.73,28.42 38.73,6.03 35.24,2.54 19.05,2.54 18.92,2.41 17.27,2.41 17.02,2.67 6.22,2.67 5.84,3.05 3.27,5.24 2.22,5.24 1.43,6.03 1.43,14.29 2.54,15.4 2.86,15.4 3.65,16.19 3.65,16.83 2.54,17.94 2.22,17.94 1.43,18.73 1.43,20.48 ARDUINO_NANO1.24
  Bottom 0.203: v39.85,58.9 42.55,61.59 42.55,70.33 41.75,71.12 36.99,71.12 RGBLED.3 | v36.83,43.02 36.83,40.48 38.73,38.58 v38.73,28.42
RGBLED_G  (via drill 0.2)
  Top 0.203: v4.6,25.4 v19.53,25.4
  Bottom 0.203: RGBLED.2 36.2,72.39 35.56,71.75 35.56,70.01 37.31,68.26 37.31,66.83 38.1,66.04 38.1,64.14 39.05,63.18 39.69,63.18 40.32,62.55 40.32,61.02 38.23,58.93 38.23,58.55 37.97,58.29 32.15,53.75 30.1,53.75 27.78,51.44 27.78,39.37 32.54,34.61 32.54,31.43 27.3,26.19 20.32,26.19 v19.53,25.4 | v4.6,25.4 3.33,24.13 ARDUINO_NANO1.23
RGBLED_R  (via drill 0.2)
  Top 0.203: v36.99,74.61 36.99,71.44 41.91,66.52 41.91,61.91 v41.08,61.09 | v39.37,42.7 39.37,37.94 32.7,31.27 v32.7,30.64 | v20.48,25.4 18.1,27.78 v4.6,27.78
  Bottom 0.203: v36.99,74.61 36.99,73.66 RGBLED.1 | v41.08,61.09 38.73,58.74 38.73,58.42 37.94,57.63 37.94,55.66 39.12,54.48 39.12,53.47 38.48,52.83 36.07,52.83 35.69,52.45 34.77,51.44 34.77,47.31 v39.37,42.7 | v32.7,30.64 27.46,25.4 v20.48,25.4 | v4.6,27.78 3.17,29.21 ARDUINO_NANO1.21
SCK
  Top 0.203: ARDUINO_NANO1.1 21.11,3.02 31.11,3.02 31.43,3.33 31.43,6.51 28.73,9.21 28.73,22.7 27.78,23.65 26.99,23.65 MCP23S17SS.12
VDD  (via drill 0.25)
  Top 0.406: v20.57,63.12 20.95,63.5 v22.86,63.5
  Bottom 0.406: 4511D.1.16 20.22,74.19 SH1.1 22.23,76.2 31.75,76.2 32.38,75.56 4511D.2.16 32.38,71.25 35.56,68.07 35.56,64.77 34.29,63.5 v22.86,63.5 | 4511D.3.16 18.41,61.21 20.32,63.12 v20.57,63.12
VSS
  Bottom 0.406: SH2.2 20.42,68.05 | 20.42,68.05 4511D.2.8 | 20.42,68.05 20.42,68.48 19.05,69.85 10.16,69.85 9.53,69.22 4511D.1.8 7.62,66.14 7.62,53.34 8.15,52.81 4511D.3.8

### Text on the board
tNames: Tanner Karbonik / Zane Johnson / Erin McFadden / Matthew Situmeang | Michael Pass | Group 28 | BME Senior Design / University of Iowa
